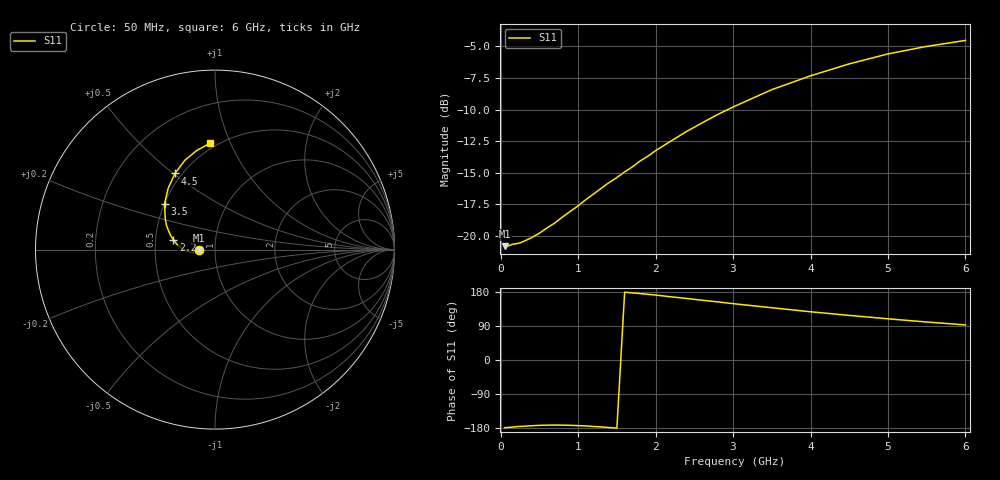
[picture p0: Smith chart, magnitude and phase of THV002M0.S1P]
! SIEMENS Discrete & RF Semiconductors
! BAS70
! Si Schottky Diode in SOT23
! IF = 2 mA
! S-Parameters:  February  1997
# GHz  S  MA  R  50
!  f  S11
! GHz  MAG  ANG
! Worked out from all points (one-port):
!   34 points, 50 MHz to 6 GHz, reference 50 ohm
!   lowest |S11| = -20.8 dB at 50 MHz (marker M1), VSWR 1.20, Z = 41.6 - j0.174 ohm
!   |S11| at or under -10 dB: start of sweep to 2.931 GHz
!   S11 on the Smith chart (normalised r, x): 50 MHz: 0.83, -0.00; 2.2 GHz: 0.62, +0.07; 3.5 GHz: 0.50, +0.30; 4.5 GHz: 0.46, +0.51; 6 GHz: 0.46, +0.84
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0.05  0.09121 -178.7
0.1  0.0914 -177.9
0.15  0.09277 -177.0
0.25  0.09394 -175.2
0.4  0.09862 -173.5
0.5  0.1027 -172.5
0.7  0.1127 -171.7
0.8  0.1191 -171.9
1  0.1317 -173.2
1.1  0.1394 -174.1
1.3  0.1547 -176.5
1.4  0.1628 -178.2
1.5  0.1704 -179.7
1.6  0.1794 178.9
1.7  0.1877 177.1
1.8  0.1981 175.3
1.9  0.2069 173.3
2  0.2177 171.4
2.2  0.2378 166.7
2.4  0.2591 162.4
2.8  0.3023 153.4
3  0.3238 148.7
3.5  0.3792 137.9
4  0.4301 127.3
4.5  0.4795 117.7
5  0.525 108.7
5.5  0.5623 100.3
6  0.5934 92.6
